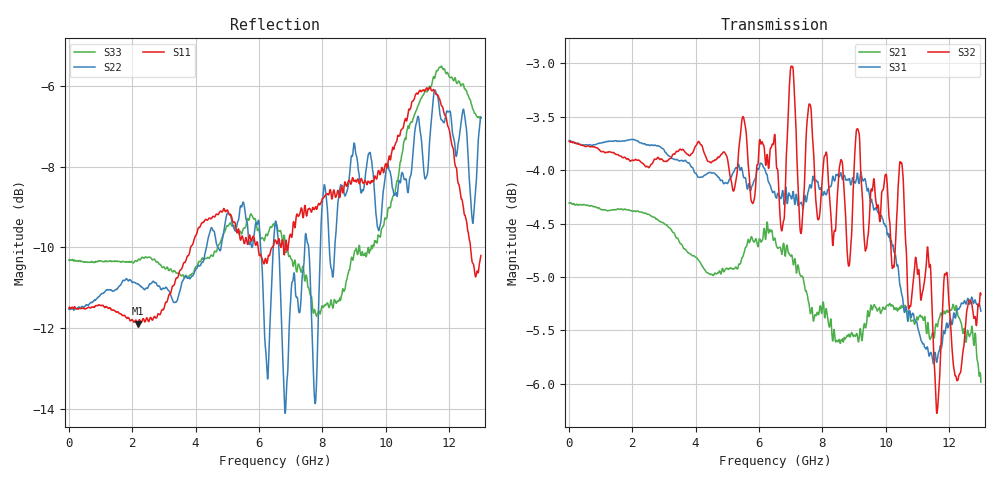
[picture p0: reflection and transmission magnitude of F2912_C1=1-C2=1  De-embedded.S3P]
! Integrated Device Technology
! Corporate Headquarters
! 6024 Silver Creek Valley Road
! San Jose, CA 95138  USA
! Phone:  1-408-284-8200
! Toll Free:  1-800-223-1366
! Webpage:  http://www.idt.com/
! Timing and RF Division
! 515 Groton Road, Suite 102
! Westford, MA 01886-6024
! Device:  F2912
! Description: High Reliability SP2T RF Switch
! Frequency:  9 kHz -  9 GHz
! Package:  4x4 mm QFN Plastic Package: 20 pin
! Ports:  3 RF, 5 DC
!  Pin  1  = GND
!  Pin  2  = GND
!  Pin  3  = RF1  =  Port 1
!  Pin  4  = GND
!  Pin  5  = GND
!  Pin  6  = GND
!  Pin  7  = GND
!  Pin  8  = RF_COM =  Port 3
!  Pin  9  = GND
!  Pin 10  = GND
!  Pin 11  = GND
!  Pin 12  = GND
!  Pin 13  = RF2  =  Port 2
!  Pin 14  = GND
!  Pin 15  = GND
!  Pin 16  = CTL2
!  Pin 17  = CTL1
!  Pin 18  = LogicCTL
!  Pin 19  = ModeCTL
!  Pin 20  = Vcc
! Logic:  3.3 V
! Mode:  2 pin control
! Voltage:  +3.30  Volts
! Current:  0.027 mA
! State:  UNDEFINED
! CTL1:  Logic HIGH
! CTL2:  Logic HIGH
! Data:  The device was measured on a F2912 evaluation board which has
!  individual transmission lines to the RF pins.  Data was collected
!  using a calibrated network analyzer.  The evaluation board was
!  de-embedded using AFR (Keysight).
!  The reference plane is the edge of the package pin.
! Misc:  Action Tracker AT0438
! Date Measured:  2018-12-14
! Date:  2018-12-14  MJV
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# Hz S dB R 50
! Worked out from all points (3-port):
!   1300 points, 10 MHz to 13 GHz, reference 50 ohm
!   strongest paths, dB at 10 MHz, 3.26 GHz, 6.51 GHz, 9.76 GHz, 13 GHz:
!     S32: -3.7, -3.9, -3.7, -4.3, -5.2
!     S31: -3.7, -3.9, -4.2, -4.4, -5.3
!     S21: -4.3, -4.6, -4.6, -5.3, -6.0
!   lowest |S11| = -11.9 dB at 2.17 GHz (marker M1), VSWR 1.68, Z = 31 + j8.34 ohm
!   |S11| at or under -10 dB: start of sweep to 3.842 GHz; 5.973 GHz to 6.409 GHz (436.6 MHz wide, 7.05 % of centre); 12.67 GHz to end of sweep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
1e7  -11.50 179.9  -4.31 -0.2  -3.74 -0.1
     -4.31 -0.2  -11.54 179.9  -3.75 -0.2
     -3.72 -0.1  -3.73 -0.1  -10.32 179.9
2.17e9  -11.89 150.4  -4.40 -20.6  -3.72 -15.5
        -4.38 -20.5  -10.91 152.7  -3.91 -14.7
        -3.73 -15.6  -3.91 -14.8  -10.33 163.9
5.48e9  -9.73 105.5  -5.32 -48.8  -4.03 -39.9
        -4.82 -49.2  -8.92 101.1  -4.08 -38.4
        -4.02 -39.7  -3.51 -38.3  -9.61 122.6
6.26e9  -10.37 105.8  -4.21 -62.0  -4.03 -46.6
        -4.49 -58.0  -13.19 106.2  -3.83 -44.2
        -4.05 -46.3  -3.85 -45.1  -9.71 132.3
6.51e9  -9.81 104.3  -4.88 -60.4  -4.25 -47.2
        -4.65 -61.5  -9.40 104.6  -3.97 -46.6
        -4.23 -47.7  -3.70 -45.9  -9.47 133.8
7.77e9  -9.02 92.1  -5.21 -79.4  -4.12 -57.1
        -5.35 -74.9  -13.87 91.7  -4.12 -57.6
        -4.10 -57.3  -4.17 -53.7  -11.59 120.6
8.04e9  -8.76 87.4  -5.48 -78.0  -4.18 -59.5
        -5.26 -78.0  -8.56 78.9  -3.97 -61.1
        -4.22 -59.4  -3.92 -61.7  -11.47 112.1
9.06e9  -8.37 69.5  -6.34 -82.0  -4.08 -70.7
        -5.54 -85.2  -7.69 75.2  -4.34 -69.5
        -4.10 -70.5  -3.67 -72.5  -10.04 85.8
1.159e10  -6.21 116.5  -5.18 -115.4  -5.60 -94.3
          -5.44 -115.5  -6.19 116.3  -5.44 -94.6
          -5.79 -94.6  -6.21 -92.1  -5.64 136.2
1.3e10  -10.20 76.9  -6.24 -150.3  -5.38 -116.6
        -5.98 -141.4  -6.77 93.6  -5.35 -109.5
        -5.32 -117.2  -5.17 -109.9  -6.80 126.8
